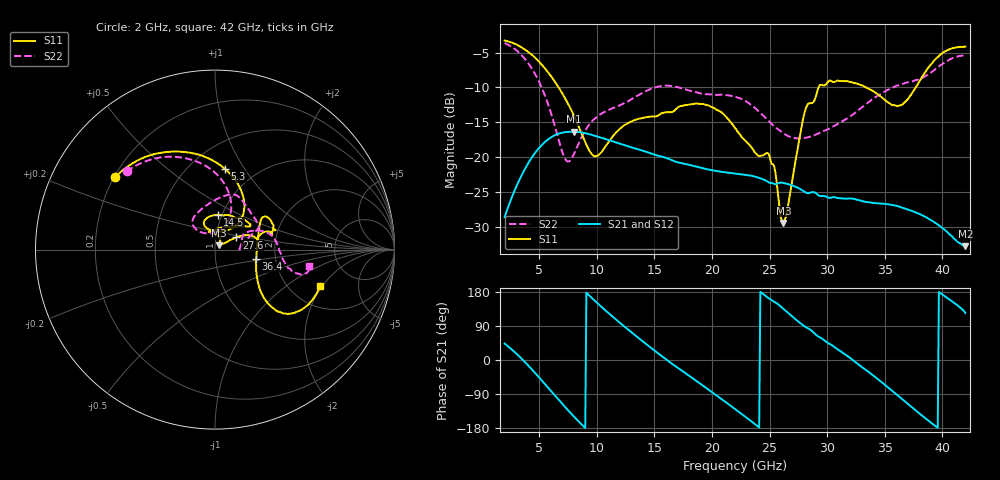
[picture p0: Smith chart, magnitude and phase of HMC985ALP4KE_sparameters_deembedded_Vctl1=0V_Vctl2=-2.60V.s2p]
!s2p File: Measurements: S11, S21, S12, S22
# GHz S dB R 50.0
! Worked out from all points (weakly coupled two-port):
!   401 points, 2 GHz to 42 GHz, reference 50 ohm
!   highest |S21| = -16.37 dB at 8 GHz (marker M1); lowest = -32.8 dB at 42 GHz (marker M2)
!   lowest |S11| = -29.5 dB at 26.2 GHz (marker M3), VSWR 1.07, Z = 52.3 + j2.57 ohm
!   |S11| at or under -10 dB: 6.684 GHz to 29.26 GHz (22.58 GHz wide, 126 % of centre); 33.38 GHz to 37.7 GHz (4.315 GHz wide, 12.1 % of centre)
!   |S22| runs from -20.6 to -3.6 dB; largest |S21 - S12| = 0.00066
!   S11 on the Smith chart (normalised r, x): 2 GHz: 0.20, +0.31; 5.3 GHz: 0.73, +0.82; 14.5 GHz: 0.95, +0.38; 27.6 GHz: 1.25, +0.17; 36.4 GHz: 1.58, -0.18; 42 GHz: 2.91, -1.90
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2  -3.26 143.8  -28.65 43.5  -28.64 43.5  -3.64 138.5
3.5  -4.29 117.2  -22.56 2.7  -22.57 2.7  -5.43 107.9
5.3  -6.89 82.8  -18.16 -56.8  -18.18 -56.8  -10.33 73.9
7.2  -11.42 53.1  -16.45 -122.6  -16.48 -122.6  -20.09 84.9
8  -14.00 48.7  -16.38 -148.7  -16.35 -148.7  -19.65 119.6
8.7  -16.71 52.6  -16.49 -170.5  -16.50 -170.5  -17.10 131.8
10  -19.87 88.9  -17.04 151.4  -17.02 151.5  -14.24 130.3
14.5  -14.23 85.8  -19.37 36.9  -19.34 37.0  -10.36 80.2
15.4  -13.96 73.6  -19.86 16.0  -19.89 15.9  -9.87 73.2
19.3  -12.42 33.9  -21.66 -69.4  -21.67 -69.5  -10.90 43.5
22  -15.81 52.2  -22.38 -129.3  -22.40 -129.4  -11.35 26.5
25  -19.91 99.0  -23.71 161.6  -23.67 161.6  -14.96 16.2
26.2  -29.46 46.8  -23.73 134.9  -23.77 134.9  -16.60 6.1
27.6  -17.31 29.9  -24.55 98.9  -24.56 98.8  -17.30 0.3
28.1  -13.27 21.0  -25.08 87.7  -25.12 87.6  -17.25 1.7
28.7  -12.24 13.0  -25.05 75.8  -25.05 75.8  -16.97 5.6
31  -9.05 23.3  -25.91 26.3  -25.90 26.2  -15.16 26.8
33.3  -9.93 34.2  -26.43 -24.8  -26.42 -24.9  -12.54 26.3
35.4  -12.27 12.0  -26.82 -75.1  -26.80 -75.1  -10.26 17.5
36.4  -12.58 -13.2  -27.21 -100.5  -27.24 -100.5  -9.54 11.7
39.5  -5.82 -43.4  -29.58 -176.4  -29.57 -176.5  -7.24 -14.5
42  -4.15 -18.9  -32.81 124.0  -32.81 123.9  -5.45 -9.8
